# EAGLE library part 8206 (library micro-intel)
MICROCOMPUTER/PERIPHERAL DEVICE
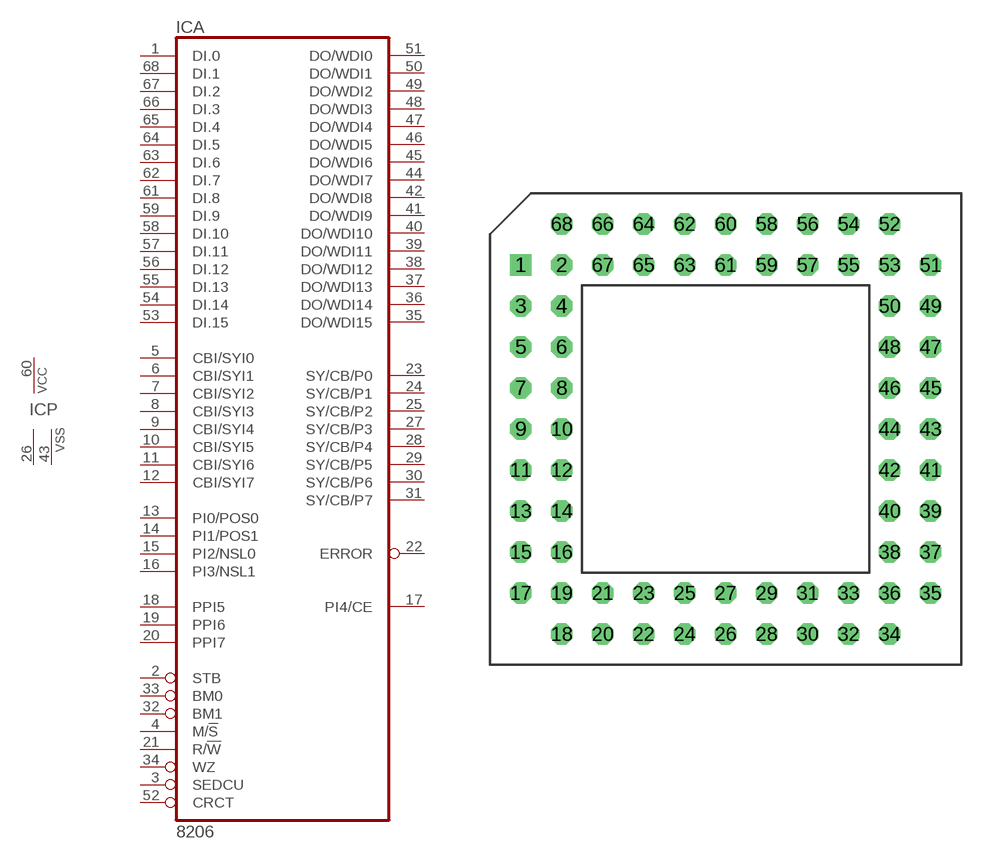
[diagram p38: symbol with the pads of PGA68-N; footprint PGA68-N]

Designator prefix IC; gates A=8206 P=PWR2VSS

## 8206 (OC_FARNELL: unknown; OC_NEWARK: unknown)  [PGA68-N]
1  A:DI.0  in
2  A:STB  in
3  A:SEDCU  in
4  A:M/!S  in
5  A:CBI/SYI0  in
6  A:CBI/SYI1  in
7  A:CBI/SYI2  in
8  A:CBI/SYI3  in
9  A:CBI/SYI4  in
10  A:CBI/SYI5  in
11  A:CBI/SYI6  in
12  A:CBI/SYI7  in
13  A:PI0/POS0  in
14  A:PI1/POS1  in
15  A:PI2/NSL0  in
16  A:PI3/NSL1  in
17  A:PI4/CE
18  A:PPI5  in
19  A:PPI6  in
20  A:PPI7  in
21  A:R/!W  in
22  A:ERROR  out
23  A:SY/CB/P0  out
24  A:SY/CB/P1  out
25  A:SY/CB/P2  out
26  P:VSS  pwr
27  A:SY/CB/P3  out
28  A:SY/CB/P4  out
29  A:SY/CB/P5  out
30  A:SY/CB/P6  out
31  A:SY/CB/P7  out
32  A:BM1  in
33  A:BM0  in
34  A:WZ  in
35  A:DO/WDI15
36  A:DO/WDI14
37  A:DO/WDI13
38  A:DO/WDI12
39  A:DO/WDI11
40  A:DO/WDI10
41  A:DO/WDI9
42  A:DO/WDI8
43  P:VSS  pwr
44  A:DO/WDI7
45  A:DO/WDI6
46  A:DO/WDI5
47  A:DO/WDI4
48  A:DO/WDI3
49  A:DO/WDI2
50  A:DO/WDI1
51  A:DO/WDI0
52  A:CRCT  in
53  A:DI.15  in
54  A:DI.14  in
55  A:DI.13  in
56  A:DI.12  in
57  A:DI.11  in
58  A:DI.10  in
59  A:DI.9  in
60  P:VCC  pwr
61  A:DI.8  in
62  A:DI.7  in
63  A:DI.6  in
64  A:DI.5  in
65  A:DI.4  in
66  A:DI.3  in
67  A:DI.2  in
68  A:DI.1  in

## Footprint PGA68-N (pad centres in mm)
Pin Grid Array
drill 0.813 square: 1 -12.7,10.16
drill 0.813 octagon: 2 -10.16,10.16; 3 -12.7,7.62; 4 -10.16,7.62; 5 -12.7,5.08; 6 -10.16,5.08; 7 -12.7,2.54; 8 -10.16,2.54; 9 -12.7,0; 10 -10.16,0; 11 -12.7,-2.54; 12 -10.16,-2.54; 13 -12.7,-5.08; 14 -10.16,-5.08; 15 -12.7,-7.62; 16 -10.16,-7.62; 17 -12.7,-10.16; 18 -10.16,-12.7; 19 -10.16,-10.16; 20 -7.62,-12.7; 21 -7.62,-10.16; 22 -5.08,-12.7; 23 -5.08,-10.16; 24 -2.54,-12.7; 25 -2.54,-10.16; 26 0,-12.7; 27 0,-10.16; 28 2.54,-12.7; 29 2.54,-10.16; 30 5.08,-12.7; 31 5.08,-10.16; 32 7.62,-12.7; 33 7.62,-10.16; 34 10.16,-12.7; 35 12.7,-10.16; 36 10.16,-10.16; 37 12.7,-7.62; 38 10.16,-7.62; 39 12.7,-5.08; 40 10.16,-5.08; 41 12.7,-2.54; 42 10.16,-2.54; 43 12.7,0; 44 10.16,0; 45 12.7,2.54; 46 10.16,2.54; 47 12.7,5.08; 48 10.16,5.08; 49 12.7,7.62; 50 10.16,7.62; 51 12.7,10.16; 52 10.16,12.7; 53 10.16,10.16; 54 7.62,12.7; 55 7.62,10.16; 56 5.08,12.7; 57 5.08,10.16; 58 2.54,12.7; 59 2.54,10.16; 60 0,12.7; 61 0,10.16; 62 -2.54,12.7; 63 -2.54,10.16; 64 -5.08,12.7; 65 -5.08,10.16; 66 -7.62,12.7; 67 -7.62,10.16; 68 -10.16,12.7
